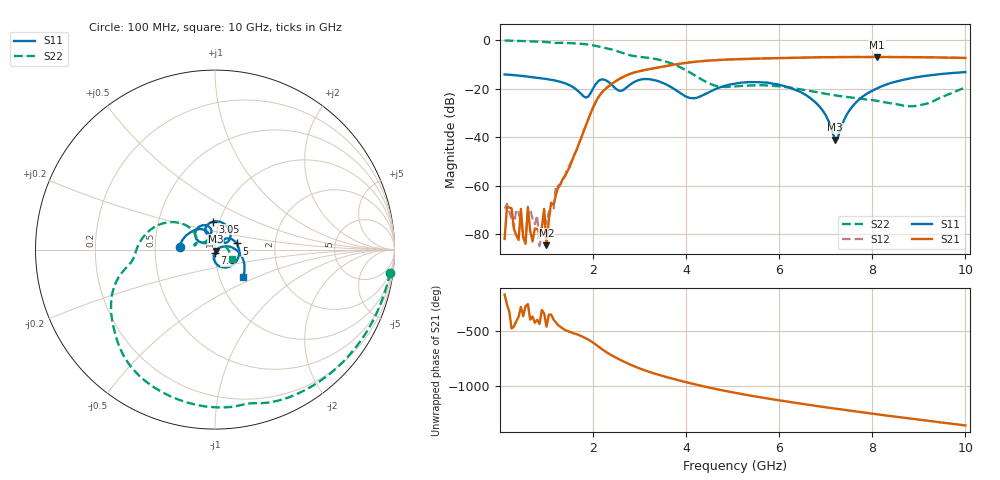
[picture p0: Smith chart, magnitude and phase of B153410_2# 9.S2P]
!  2-Port S-parameters saved by WinCal
! VAR MeasName=S-Parameters (CALIBRATED_DATA) read from VNA (N5245A)
! VAR MeasDate=2016-12-23 9:59:48
! VAR NAME=B153410_2# 9
! VAR FILENAME=B153410_2# 9.S2P
! VAR DATE=2016-12-23 9:59:48
! VAR PHYS_PORTS=1,2
# Hz S DB R 50
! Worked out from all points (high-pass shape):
!   199 points, 100 MHz to 10 GHz, reference 50 ohm
!   highest |S21| = -6.92 dB at 8.1 GHz (marker M1); lowest = -84.5 dB at 1 GHz (marker M2)
!   |S21| within 3 dB of the highest: 3.795 GHz to end of sweep
!   lowest |S11| = -40.9 dB at 7.2 GHz (marker M3), VSWR 1.02, Z = 50.5 - j0.73 ohm
!   |S11| at or under -10 dB: start of sweep to end of sweep
!   |S22| runs from -27.2 to -0.1 dB; largest |S21 - S12| = 0.0032
!   S11 on the Smith chart (normalised r, x): 100 MHz: 0.67, +0.02; 3.05 GHz: 0.93, +0.30; 5 GHz: 1.27, +0.09; 7.1 GHz: 1.00, -0.03; 10 GHz: 1.29, -0.42
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1e8  -14.14 175.2  -81.85 -165.8  -69.41 -45.6  -0.13 -7.5
1.5e8  -14.18 172.7  -68.77 104.2  -67.39 123.6  -0.18 -10.9
3.5e8  -14.49 163.1  -80.28 -50.6  -69.71 34.1  -0.30 -24.3
4.5e8  -14.67 159.0  -69.46 81.2  -74.93 110.9  -0.36 -31.0
5.5e8  -14.90 154.7  -83.84 88.4  -81.78 -6.9  -0.43 -37.6
6e8  -15.02 152.8  -68.67 107.0  -70.66 -78.7  -0.45 -40.8
7e8  -15.29 149.2  -82.85 -7.1  -73.49 14.0  -0.52 -47.4
9.5e8  -15.88 139.2  -69.48 20.0  -71.77 12.0  -0.72 -63.8
1e9  -16.01 137.4  -84.47 -99.3  -75.39 19.5  -0.79 -67.1
1.1e9  -16.32 133.2  -66.91 10.7  -69.89 20.4  -0.98 -73.4
1.75e9  -22.27 115.4  -40.14 173.2  -39.91 172.8  -1.52 -113.5
2.2e9  -16.15 125.9  -21.32 51.6  -21.33 51.8  -2.96 -142.6
3.05e9  -16.14 94.6  -12.55 -130.0  -12.55 -130.0  -6.99 -176.6
3.4e9  -16.87 59.3  -11.25 -178.9  -11.25 -178.8  -8.00 168.2
5e9  -18.05 15.8  -7.91 19.0  -7.91 19.1  -19.13 165.6
5.05e9  -17.87 12.3  -7.88 14.9  -7.89 15.1  -19.05 166.8
6.7e9  -24.36 -93.6  -7.10 -99.1  -7.10 -99.1  -21.03 153.0
7.1e9  -35.19 -92.7  -7.01 -123.5  -7.01 -123.4  -22.40 151.1
7.2e9  -40.93 -53.6  -6.99 -129.6  -6.98 -129.4  -22.73 150.9
8.1e9  -19.86 5.1  -6.92 178.5  -6.94 178.7  -24.99 135.1
8.35e9  -17.94 -3.7  -6.96 164.6  -6.95 164.9  -25.87 122.1
1e10  -13.16 -44.6  -7.33 76.4  -7.33 76.8  -19.51 -28.4
